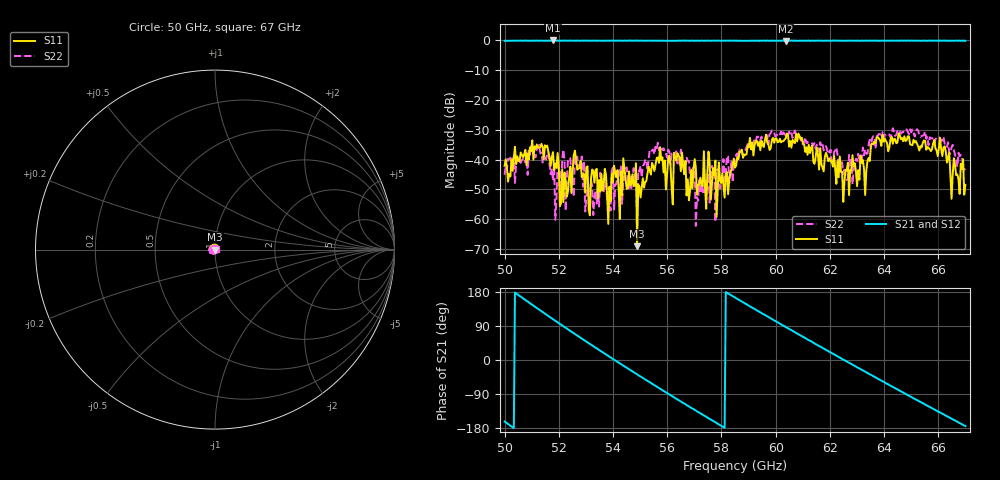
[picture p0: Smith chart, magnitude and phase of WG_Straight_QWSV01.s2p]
!Agilent Technologies,E8361A,US42410132,A.06.03.05
!Agilent E8361A: A.06.03.05
!Date: Friday, July 11, 2008 15:37:39
!Correction: S11(Full 2 Port(1,2)) S21(Full 2 Port(1,2)) S12(Full 2 Port(1,2)) S22(Full 2 Port(1,2))
!S2P File: Measurements: S11, S21, S12, S22:
# Hz S  MA  R 50
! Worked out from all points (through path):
!   401 points, 50 GHz to 67 GHz, reference 50 ohm
!   highest |S21| = -0.01 dB at 51.78 GHz (marker M1); lowest = -0.2 dB at 60.37 GHz (marker M2)
!   lowest |S11| = -69.1 dB at 54.89 GHz (marker M3), VSWR 1.00, Z = 50 + j0.0345 ohm
!   |S11| at or under -10 dB: start of sweep to end of sweep
!   |S22| runs from -62.3 to -29.5 dB; largest |S21 - S12| = 0.019
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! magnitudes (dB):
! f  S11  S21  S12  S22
! 50 GHz  -42.1  -0.1  0.0  -45.1
! 51.27 GHz  -36.0  -0.1  -0.1  -35.1
! 51.78 GHz  -37.5  0.0  -0.1  -47.1
! 52.12 GHz  -43.3  0.0  -0.1  -39.6
! 52.85 GHz  -45.9  0.0  -0.1  -39.0
! 53.06 GHz  -42.3  -0.1  -0.1  -49.0
! 53.31 GHz  -47.8  -0.1  0.0  -52.5
! 53.83 GHz  -61.6  -0.1  0.0  -50.7
! 54.08 GHz  -44.4  -0.1  -0.1  -48.5
! 54.89 GHz  -69.1  -0.1  0.0  -58.9
! 55.7 GHz  -41.1  -0.1  -0.1  -37.0
! 56.46 GHz  -39.3  -0.1  -0.1  -41.7
! 56.76 GHz  -46.7  -0.1  -0.1  -40.4
! 57.14 GHz  -48.5  -0.1  -0.1  -53.9
! 58.16 GHz  -44.9  -0.1  -0.1  -44.2
! 58.5 GHz  -42.7  -0.1  -0.1  -40.7
! 60.37 GHz  -32.9  -0.2  -0.1  -31.9
! 61.35 GHz  -35.2  -0.1  -0.1  -34.5
! 62.58 GHz  -43.6  -0.1  -0.1  -45.6
! 64.19 GHz  -35.9  -0.1  -0.1  -31.6
! 66.15 GHz  -38.9  -0.1  -0.1  -33.7
! 67 GHz  -48.5  -0.1  -0.2  -43.1
